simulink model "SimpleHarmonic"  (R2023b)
settings: Solver=VariableStepAuto  StartTime=0.0  StopTime=10.0  RelTol=1e-3

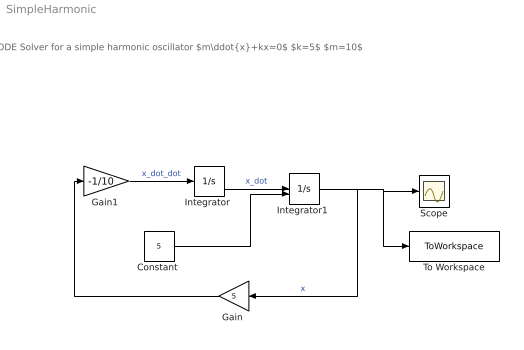
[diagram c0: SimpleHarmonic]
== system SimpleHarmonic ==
  note: ODE Solver for a simple harmonic oscillator $m\ddot{x}+kx=0$ $k=5$ $m=10$
  "Constant " : Constant  Value=5
  "Gain " : Gain  Gain=5
  "Gain1 " : Gain  Gain=-1/10
  "Integrator " : Integrator
  "Integrator1 " : Integrator  InitialConditionSource=external
  Scope : Scope
  To Workspace : ToWorkspace  VariableName=sol  SaveFormat=Timeseries  SampleTime=-1
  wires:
  "Integrator "/1 -> "Integrator1 "/1  "x_dot"
  "Integrator1 "/1 -> To Workspace/1, Scope/1, "Gain "/1  "x"
  "Gain1 "/1 -> "Integrator "/1  "x_dot_dot"
  "Gain "/1 -> "Gain1 "/1
  "Constant "/1 -> "Integrator1 "/2
